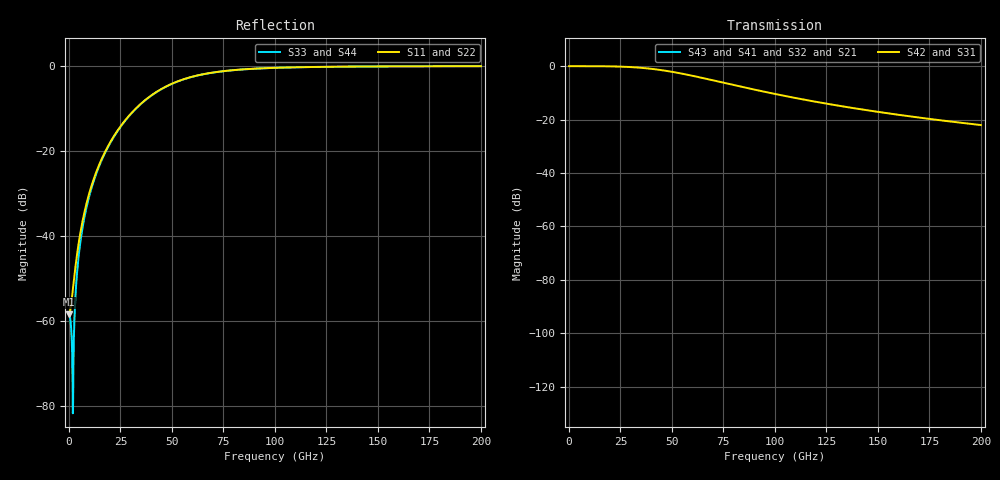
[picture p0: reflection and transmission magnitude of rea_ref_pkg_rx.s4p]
! Created with skrf 1.10.0 (http://scikit-rf.org).
# Hz S RI R 50.0
!freq ReS11 ImS11 ReS12 ImS12 ReS13 ImS13
! ReS14 ImS14
! ReS21 ImS21 ReS22 ImS22 ReS23 ImS23
! ReS24 ImS24
! ReS31 ImS31 ReS32 ImS32 ReS33 ImS33
! ReS34 ImS34
! ReS41 ImS41 ReS42 ImS42 ReS43 ImS43
! ReS44 ImS44
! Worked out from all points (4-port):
!   2000 points, 100 MHz to 200 GHz, reference 50 ohm
!   strongest paths, dB at 100 MHz, 50.1 GHz, 100.1 GHz, 150.1 GHz, 200 GHz:
!     S42: 0.0, -2.1, -10.4, -17.1, -22.1
!     S31: 0.0, -2.1, -10.4, -17.1, -22.1
!     S43: -, -, -, -, -
!     S41: -, -, -, -, -
!     S32: -, -, -, -, -
!     S21: -, -, -, -, -
!   lowest |S11| = -58.4 dB at 100 MHz (marker M1), VSWR 1.00, Z = 50.1 - j0.000605 ohm
!   |S11| at or under -10 dB: start of sweep to 32.45 GHz
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1e8  0.0012 -6.03e-06  0 0  0.9988 -0.00251  0 0
     0 0  0.0012 -6.03e-06  0 0  0.9988 -0.00251
     0.9988 -0.00251  0 0  0.0012 7.92e-09  0 0
     0 0  0.9988 -0.00251  0 0  0.0012 7.92e-09
2e9  0.00245 -0.000184  0 0  0.9975 -0.0502  0 0
     0 0  0.00245 -0.000184  0 0  0.9975 -0.0502
     0.9975 -0.0502  0 0  -6.01e-05 6.33e-05  0 0
     0 0  0.9975 -0.0502  0 0  -6.01e-05 6.33e-05
5.9e9  0.012 -0.00198  0 0  0.9877 -0.1481  0 0
       0 0  0.012 -0.00198  0 0  0.9877 -0.1481
       0.9877 -0.1481  0 0  -0.00965 0.00163  0 0
       0 0  0.9877 -0.1481  0 0  -0.00965 0.00163
1.44e10  0.0618 -0.0244  0 0  0.9293 -0.3599  0 0
         0 0  0.0618 -0.0244  0 0  0.9293 -0.3599
         0.9293 -0.3599  0 0  -0.0596 0.0235  0 0
         0 0  0.9293 -0.3599  0 0  -0.0596 0.0235
4.35e10  0.1765 -0.482  0 0  0.2965 -0.8043  0 0
         0 0  0.1765 -0.482  0 0  0.2965 -0.8043
         0.2965 -0.8043  0 0  -0.1758 0.4801  0 0
         0 0  0.2965 -0.8043  0 0  -0.1758 0.4801
7.86e10  -0.3862 -0.8016  0 0  -0.1973 -0.4108  0 0
         0 0  -0.3862 -0.8016  0 0  -0.1973 -0.4108
         -0.1973 -0.4108  0 0  0.3858 0.8006  0 0
         0 0  -0.1973 -0.4108  0 0  0.3858 0.8006
2e11  -0.9151 -0.3954  0 0  -0.0724 -0.0313  0 0
      0 0  -0.9151 -0.3954  0 0  -0.0724 -0.0313
      -0.0724 -0.0313  0 0  0.9149 0.3953  0 0
      0 0  -0.0724 -0.0313  0 0  0.9149 0.3953
